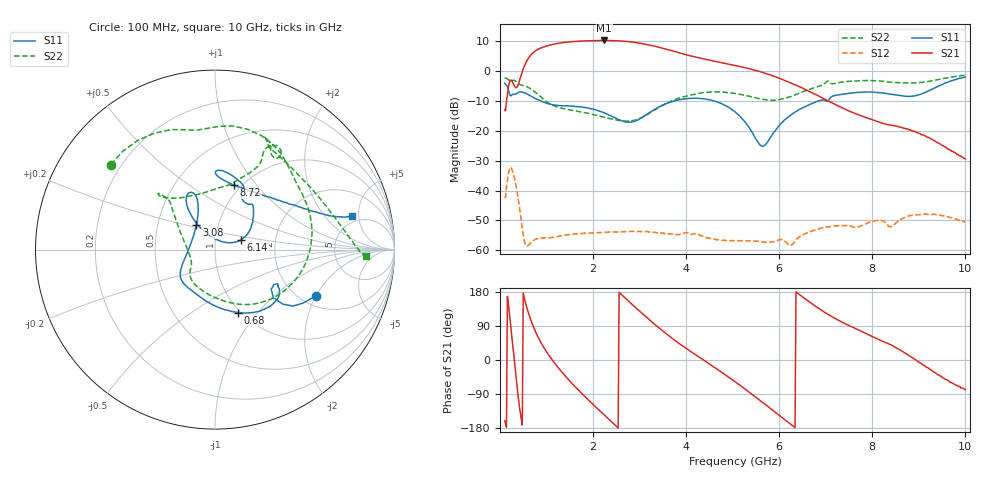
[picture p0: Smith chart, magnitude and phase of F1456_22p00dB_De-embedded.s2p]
! Integrated Device Technology
! Corporate Headquarters
! 6024 Silver Creek Valley Road
! San Jose, CA 95138  USA
! Phone:  1-408-284-8200
! Toll Free:  1-800-223-1366
! Webpage:  http://www.idt.com/
! Timing and RF Division
! 515 Groton Road, Suite 102
! Westford, MA 01886-6024
! Device:  F1456
! Description: 6-bit 0.5 dB Transmit Variable Gain Amplifier
! Frequency:  2100.0 -  2950.00 MHz
! Package:  6x6 mm Thin QFN Plastic Package: 28 pin
! State:  44
! Atten State:  22.0 dB
! Voltage:  +5.00 Volts
! Current:  216.982 mA
! Data:  The device was measured on a the F1455 evaluation board which has
!  individual transmission lines to the RF pins.  Data was collected
!  using a calibrated network analyzer.  The evaluation board was
!  de-embedded using a TRL calibration technique.
!  The reference plane is the edge of the package pin.
!  Pin  1 = CSb
!  Pin  2 = DATA
!  Pin  3 = CLK
!  Pin  4 = RSET
!  Pin  5 = GND
!  Pin  6 = RFIN  = Port 1
!  Pin  7 = GND
!  Pin  8 = NC
!  Pin  9 = NC
!  Pin 10 = NC
!  Pin 11 = NC
!  Pin 12 = NC
!  Pin 13 = NC
!  Pin 14 = /STBY
!  Pin 15 = GND
!  Pin 16 = RFOUT  = Port 2
!  Pin 17 = GND
!  Pin 18 = NC
!  Pin 19 = NC
!  Pin 20 = NC
!  Pin 21 = GND
!  Pin 22 = NC
!  Pin 23 = GND
!  Pin 24 = NC
!  Pin 25 = NC
!  Pin 26 = NC
!  Pin 27 = GND
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# GHz S dB R 50
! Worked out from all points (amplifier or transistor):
!   496 points, 100 MHz to 10 GHz, reference 50 ohm
!   highest |S21| = 10.1 dB at 2.24 GHz (marker M1)
!   |S21| within 3 dB of that: 810.7 MHz to 3.594 GHz (2.784 GHz wide, 126 % of centre)
!   unconditionally stable (mu >= 1): start of sweep to end of sweep
!   at 1.74 GHz: K = 75.12, MAG = 10.4 dB, |S12| = -54.4 dB
!   at 5.06 GHz: K = 221.79, MAG = 2.8 dB, |S12| = -56.7 dB
!   at 10 GHz: K = 543.49, MAG = -19.8 dB, |S12| = -50.5 dB
!   S11 on the Smith chart (normalised r, x): 100 MHz: 2.37, -2.01; 680 MHz: 0.97, -0.79; 3.08 GHz: 0.78, +0.22; 6.14 GHz: 1.33, +0.15; 8.72 GHz: 0.93, +0.77; 10 GHz: 4.18, +4.12
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0.1  -4.15 -24.9  -13.08 -160.2  -42.33 49.4  -2.53 140.8
0.22  -8.33 -35.2  -3.16 103.0  -32.22 -51.3  -3.44 99.1
0.3  -7.84 -30.3  -4.75 11.1  -35.18 -135.8  -3.17 74.8
0.42  -7.08 -37.2  -3.26 -125.3  -45.81 139.8  -4.57 41.2
0.54  -7.43 -53.7  2.13 155.2  -57.76 135.8  -5.09 15.1
0.68  -8.58 -70.3  5.54 100.0  -57.15 144.6  -6.21 -16.9
0.86  -9.96 -88.4  7.50 50.6  -55.87 111.8  -8.50 -53.4
1.16  -11.42 -113.0  8.89 -5.7  -55.60 76.3  -11.70 -93.7
1.48  -11.76 -130.1  9.64 -52.8  -54.74 52.6  -13.00 -119.7
1.76  -12.11 -140.5  9.93 -88.6  -54.34 36.2  -13.78 -132.3
2.24  -14.04 -155.9  10.13 -145.0  -53.96 14.3  -15.50 -143.2
2.64  -16.85 175.9  9.91 169.3  -53.77 -2.5  -16.76 -157.9
3.08  -15.33 127.4  9.01 120.0  -53.78 -23.0  -15.32 168.5
3.4  -12.22 112.6  7.92 86.3  -54.07 -37.4  -12.43 148.1
4.08  -9.22 112.7  5.03 24.0  -54.58 -68.5  -8.19 133.2
5.06  -13.83 125.3  1.76 -58.0  -56.74 -117.0  -7.58 135.2
5.64  -25.22 68.8  -0.53 -111.5  -57.15 -156.5  -9.52 118.1
6.14  -16.10 20.9  -3.39 -159.6  -57.18 167.1  -9.07 83.3
6.7  -10.95 41.1  -7.28 148.6  -53.53 147.9  -5.91 63.5
8.36  -7.70 88.3  -18.09 42.4  -52.00 68.8  -3.77 62.5
8.72  -8.54 73.5  -19.40 17.0  -48.80 68.2  -4.06 50.3
10  -2.09 13.9  -29.46 -77.9  -50.49 -23.0  -1.46 -2.6
